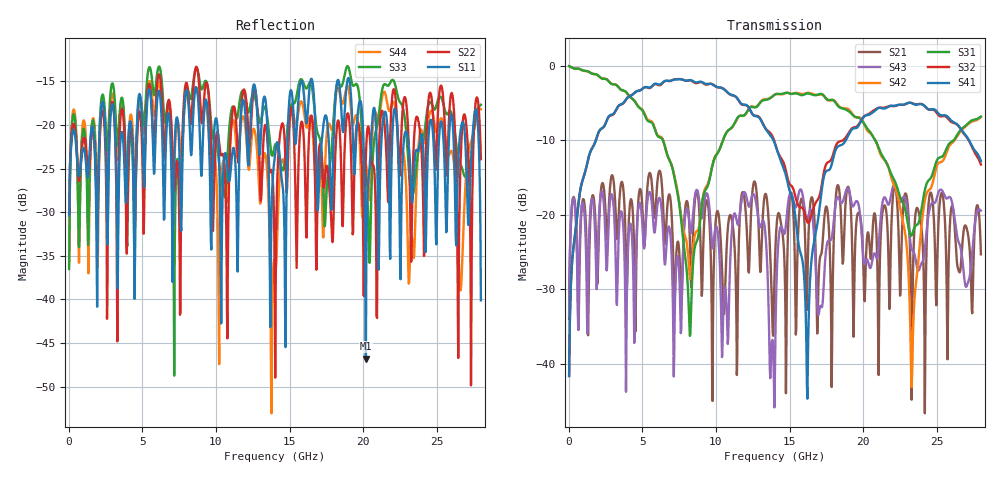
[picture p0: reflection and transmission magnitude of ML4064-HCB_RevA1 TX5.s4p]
! TOUCHSTONE file generated by CST DESIGN STUDIO
! Date and time: Wed Aug 26 10:54:55 2020
! Project name:  Project name: C:\Users\Simulation2\Temp\DE66\Untitled_0.cst
! Tree item: Tasks\SPara1\S-Parameters
# GHz S MA R 50
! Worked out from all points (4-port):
!   1000 points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, 28 MHz to 28 GHz, reference 50 ohm
!   strongest paths, dB at 28 MHz, 7.028 GHz, 14.03 GHz, 21.03 GHz, 28 GHz:
!     S41: -41.6, -1.9, -10.6, -5.7, -12.8
!     S32: -41.6, -1.9, -10.5, -5.6, -13.3
!     S31: -0.1, -13.6, -3.8, -10.9, -6.8
!     S42: -0.1, -13.6, -3.8, -11.0, -6.9
!     S43: -33.5, -27.6, -38.0, -24.8, -19.4
!     S21: -34.0, -21.4, -25.2, -37.9, -25.3
!   lowest |S11| = -46.8 dB at 20.19 GHz (marker M1), VSWR 1.01, Z = 50.2 + j0.396 ohm
!   |S11| at or under -10 dB: start of sweep to end of sweep
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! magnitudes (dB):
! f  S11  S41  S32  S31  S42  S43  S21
! 28 MHz  -30.4  -41.6  -41.6  -0.1  -0.1  -33.5  -34.0
! 8.232 GHz  -20.7  -1.9  -2.0  -36.2  -28.3  -21.7  -23.4
! 13.83 GHz  -27.1  -9.7  -9.4  -4.1  -4.1  -36.8  -33.9
! 16.21 GHz  -19.1  -44.6  -21.0  -3.7  -3.6  -20.6  -29.5
! 20.19 GHz  -46.8  -6.7  -6.6  -8.2  -8.4  -26.1  -26.1
! 23.32 GHz  -28.9  -5.1  -5.0  -22.6  -41.2  -24.7  -39.8
! 28 GHz  -40.1  -12.8  -13.3  -6.8  -6.9  -19.4  -25.3
